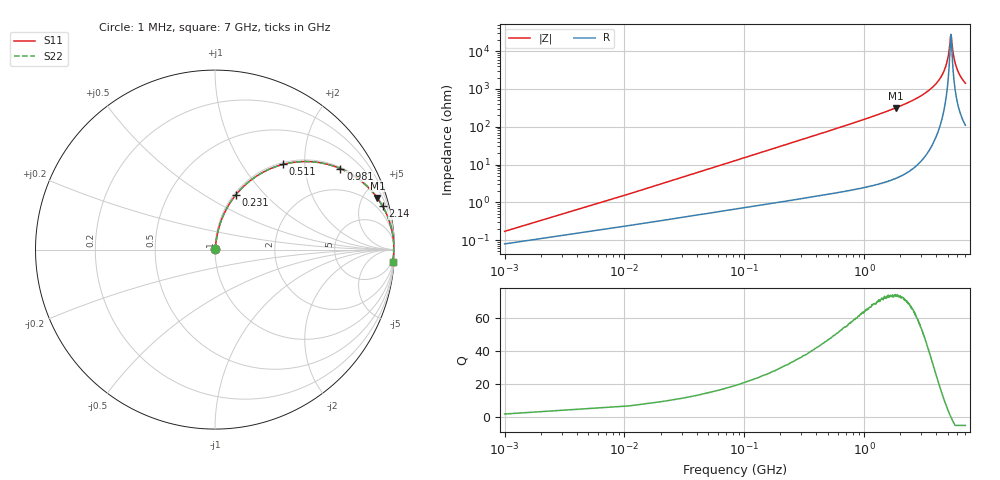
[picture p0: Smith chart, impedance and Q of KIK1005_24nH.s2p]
!version-3
!date-01.2023
!Series
# MHz S RI R 50
!Freq ReS11 ImS11 ReS21 ImS21 ReS12 ImS12 ReS22 ImS22
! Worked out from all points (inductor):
!   701 points, 1 MHz to 7 GHz, reference 50 ohm
!   read as one part in series: L = 24 nH near 31 MHz
!   highest Q = 73.4 at 1.83 GHz (marker M1), where L = 27.3 nH
!   self-resonance near 5.3 GHz
!   S11 on the Smith chart (normalised r, x): 1 MHz: 1.00, +0.00; 231 MHz: 1.02, +0.70; 511 MHz: 1.03, +1.56; 981 MHz: 1.05, +3.06; 2.14 GHz: 1.11, +7.71; 7 GHz: 3, -28
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1  0.000786 0.00151  0.9992 -0.00151  0.9992 -0.00151  0.000786 0.00151
41  0.00837 0.061  0.9916 -0.061  0.9916 -0.061  0.00837 0.061
61  0.0139 0.0902  0.9861 -0.0902  0.9861 -0.0902  0.0139 0.0902
131  0.0449 0.1872  0.9551 -0.1872  0.9551 -0.1872  0.0449 0.1872
231  0.1162 0.3051  0.8838 -0.3051  0.8838 -0.3051  0.1162 0.3051
351  0.2262 0.4058  0.7738 -0.4058  0.7738 -0.4058  0.2262 0.4058
511  0.3795 0.4748  0.6205 -0.4748  0.6205 -0.4748  0.3795 0.4748
981  0.6983 0.4511  0.3017 -0.4511  0.3017 -0.4511  0.6983 0.4511
1170  0.7717 0.4124  0.2283 -0.4124  0.2283 -0.4124  0.7717 0.4124
1830  0.9045 0.2872  0.0955 -0.2872  0.0955 -0.2872  0.9045 0.2872
2140  0.9341 0.2413  0.0659 -0.2413  0.0659 -0.2413  0.9341 0.2413
2340  0.9477 0.2154  0.0523 -0.2154  0.0523 -0.2154  0.9477 0.2154
3510  0.9862 0.1043  0.0138 -0.1043  0.0138 -0.1043  0.9862 0.1043
4190  0.9936 0.0589  0.00639 -0.0589  0.00639 -0.0589  0.9936 0.0589
4670  0.9958 0.0316  0.00415 -0.0316  0.00415 -0.0316  0.9958 0.0316
5020  0.9964 0.0136  0.00357 -0.0136  0.00357 -0.0136  0.9964 0.0136
5300  0.9964 0.000151  0.0036 -0.000151  0.0036 -0.000151  0.9964 0.000151
5340  0.9964 -0.00171  0.00364 0.00171  0.00364 0.00171  0.9964 -0.00171
5560  0.996 -0.0117  0.00396 0.0117  0.00396 0.0117  0.996 -0.0117
5840  0.9953 -0.0239  0.00466 0.0239  0.00466 0.0239  0.9953 -0.0239
6320  0.9935 -0.0435  0.0065 0.0435  0.0065 0.0435  0.9935 -0.0435
7000  0.9898 -0.0691  0.0102 0.0691  0.0102 0.0691  0.9898 -0.0691
